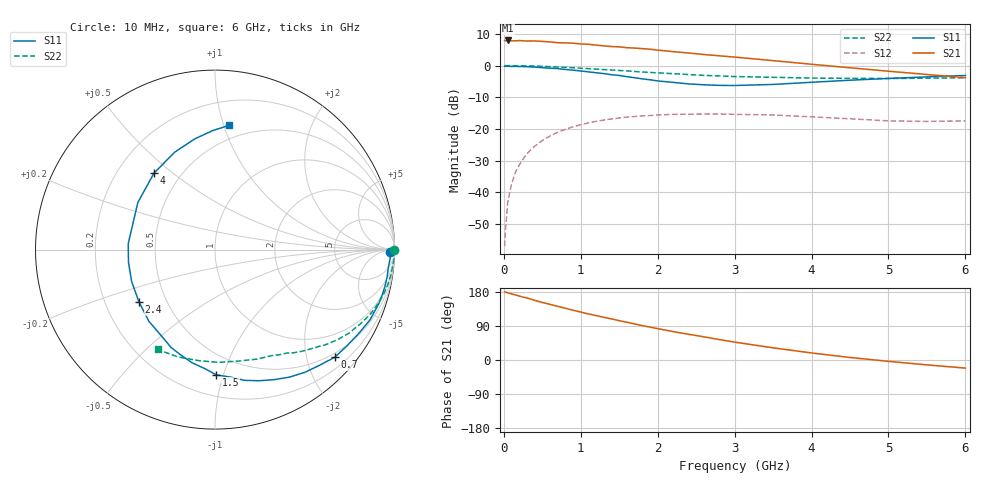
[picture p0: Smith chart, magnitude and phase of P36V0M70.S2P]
! SIEMENS Small Signal Semiconductors
! BFP181
! Si NPN RF Bipolar Junction Transistor in SOT143
! VCE = 6 V  IC = 0.7 mA
! Common Emitter S-Parameters:  March  1996
# GHz  S  MA  R  50
!  f  S11  S21  S12  S22
! GHz  MAG  ANG  MAG  ANG  MAG  ANG  MAG  ANG
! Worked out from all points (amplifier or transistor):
!   36 points, 10 MHz to 6 GHz, reference 50 ohm
!   highest |S21| = 7.9 dB at 50 MHz (marker M1)
!   |S21| within 3 dB of that: start of sweep to 1.984 GHz
!   unconditionally stable (mu >= 1): 3.618 GHz to end of sweep
!   at 250 MHz: K = 0.08, MSG = 18.7 dB, |S12| = -29.6 dB
!   at 1.4 GHz: K = 0.44, MSG = 11.4 dB, |S12| = -16.9 dB
!   at 6 GHz: K = 1.36, MAG = 3.3 dB, |S12| = -17.5 dB
!   S11 on the Smith chart (normalised r, x): 10 MHz: 67, -34; 700 MHz: 0.42, -2.55; 1.5 GHz: 0.35, -0.95; 2.4 GHz: 0.35, -0.27; 4 GHz: 0.36, +0.43; 6 GHz: 0.39, +1.04
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0.01  0.9765 -0.7  2.492 179.7  0.0014 84.1  0.9988 -0.2
0.02  0.9738 -1.1  2.467 179.4  0.0024 88.7  0.9977 -0.6
0.05  0.977 -3.0  2.496 177.2  0.0068 89.2  0.9965 -1.5
0.1  0.9707 -6.0  2.466 174.5  0.0135 84.9  0.9994 -2.9
0.15  0.9711 -9.0  2.459 171.8  0.0205 83.0  0.9956 -4.3
0.2  0.9687 -12.1  2.487 168.8  0.0268 81.5  0.9935 -5.8
0.3  0.961 -18.3  2.445 163.8  0.0406 77.6  0.989 -8.7
0.4  0.9481 -24.4  2.451 157.5  0.0531 73.4  0.9827 -11.5
0.5  0.9265 -30.5  2.412 151.8  0.0655 68.7  0.9729 -14.4
0.7  0.8973 -41.9  2.301 141.6  0.0884 61.3  0.9506 -19.7
0.9  0.847 -53.9  2.258 131.3  0.1079 53.4  0.9237 -24.7
1.1  0.7957 -65.6  2.174 121.5  0.1244 46.6  0.8946 -29.3
1.5  0.6979 -89.4  1.978 103.8  0.1487 34.3  0.8366 -37.6
1.9  0.5973 -114.3  1.816 86.8  0.1627 23.7  0.779 -44.7
2.2  0.5434 -132.7  1.661 75.0  0.1695 17.0  0.7457 -49.4
2.4  0.5139 -145.6  1.581 67.9  0.1708 12.9  0.7227 -52.7
3  0.4846 176.0  1.362 47.2  0.1697 2.6  0.6711 -61.5
3.5  0.5036 148.6  1.198 32.1  0.1657 -3.7  0.6532 -69.1
4  0.5449 128.6  1.05 18.6  0.155 -8.2  0.6348 -78.1
4.5  0.5874 112.5  0.923 6.6  0.1442 -10.8  0.6288 -88.1
5.5  0.6628 91.2  0.723 -12.9  0.1312 -7.2  0.6326 -109.0
6  0.6974 83.4  0.644 -21.4  0.1337 -4.6  0.6419 -119.9
